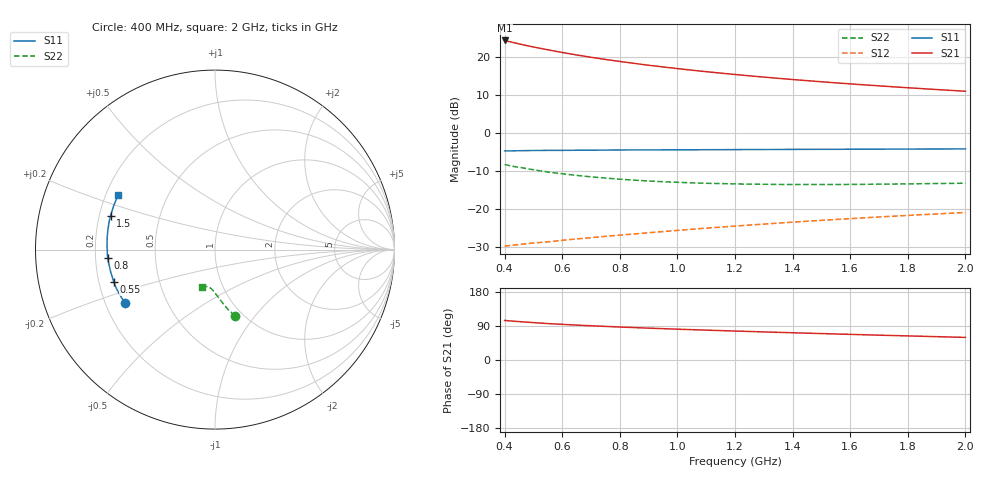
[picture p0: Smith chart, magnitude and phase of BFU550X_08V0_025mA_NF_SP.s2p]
! Filename:  P:\Prog\Test\Noise\ATS_data\Testdata_Net\BFU550X attenuator noise\BFU550X_APG2013_44_C05_08p0V_025mA_NF_CM01_D.sf
! Date/Time: Fri 26/Jul/2013 14:34:24
! BFU550X_APG2013_44_C05_08p0V_1to35mA_NF_CM01_Bias7_R.sf
! Noise Parameter Data File
! BFU550X_APG2013_44_C05_08p0V_1to35mA_NF_CM01
! Date/time: Mon Jul 22 10:19:05 2013
! VAR V_out= 8.001000
! VAR I_out= 24.995000
! VAR V_in= 0.796900
! VAR I_in= 0.264750
! Device data file deembeded for feedlines and parallel
! Original file: \BFU550X attenuator noise\BFU550X_APG2013_44_C05_08p0V_025mA_NF_CM01_R.sf
! Feed-files: PR005V01_100713_Feed1.s2p, PR005V01_100713_Feed2.s2p
! Parallel-file: PR005V01_100713_Par.s2p
# MHz S MA R 50
!  Freq-MHz  S11-mag  S11-arg  S21-mag  S21-arg  S12-mag  S12-arg  S22-mag  S22-arg
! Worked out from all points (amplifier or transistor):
!   37 points, 400 MHz to 2 GHz, reference 50 ohm
!   highest |S21| = 24.3 dB at 400 MHz (marker M1)
!   |S21| within 3 dB of that: start of sweep to 588.9 MHz
!   unconditionally stable (mu >= 1): 1.44 GHz to end of sweep
!   at 500 MHz: K = 0.66, MSG = 25.8 dB, |S12| = -28.9 dB
!   at 1.1 GHz: K = 0.95, MSG = 20.6 dB, |S12| = -25.0 dB
!   at 2 GHz: K = 1.04, MAG = 14.7 dB, |S12| = -20.9 dB
!   lowest NFmin = 1.10 dB at 480 MHz
!   S11 on the Smith chart (normalised r, x): 400 MHz: 0.28, -0.26; 550 MHz: 0.26, -0.15; 800 MHz: 0.25, -0.04; 1.5 GHz: 0.25, +0.15; 2 GHz: 0.25, +0.25
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400  0.5833 -149.1  16.48 104.3  0.03264 47.8  0.3859 -73.5
420  0.5829 -151.1  15.78 103.1  0.03332 48.1  0.3719 -74.8
440  0.5857 -153.0  15.16 101.9  0.03398 48.2  0.3593 -75.7
460  0.5869 -154.8  14.57 100.8  0.03465 48.3  0.3505 -76.9
500  0.5901 -158.1  13.53 98.7  0.03588 48.6  0.3301 -78.8
550  0.5922 -162.1  12.42 96.2  0.0372 49.4  0.3075 -81.0
600  0.5922 -165.1  11.46 94.1  0.03898 50.1  0.292 -82.8
650  0.5946 -168.1  10.62 92.1  0.04061 50.7  0.2777 -84.5
700  0.5953 -170.7  9.908 90.3  0.04222 51.5  0.2662 -86.0
750  0.5976 -173.1  9.278 88.7  0.04394 52.0  0.2563 -87.5
800  0.5995 -175.3  8.728 87.0  0.04559 52.6  0.2478 -88.9
850  0.6005 -177.5  8.235 85.5  0.0472 53.3  0.2405 -90.2
900  0.6004 -179.5  7.789 84.1  0.04899 53.9  0.2345 -91.4
950  0.6018 178.7  7.395 82.7  0.05075 54.4  0.2293 -92.5
1050  0.6031 175.2  6.706 80.1  0.05441 55.3  0.2217 -94.6
1100  0.6042 173.5  6.408 78.8  0.05628 55.6  0.2188 -95.5
1200  0.6062 170.4  5.885 76.4  0.05992 56.2  0.2148 -97.4
1350  0.6091 166.1  5.239 73.0  0.06557 56.9  0.2112 -100.0
1500  0.6113 162.1  4.722 69.7  0.0713 57.2  0.211 -102.4
1600  0.613 159.6  4.428 67.6  0.07504 57.3  0.2113 -103.8
1750  0.6151 155.9  4.052 64.6  0.08085 57.4  0.2139 -106.1
2000  0.6195 150.4  3.544 59.6  0.09038 57.1  0.2195 -109.5
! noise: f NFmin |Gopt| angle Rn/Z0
400  1.211  0.2937  -175.5  0.08
460  1.155  0.3332  -173.7  0.0681
600  1.169  0.3283  -172.3  0.0715
800  1.185  0.3507  -169.2  0.0676
1000  1.214  0.371  -166.3  0.0647
1200  1.239  0.3929  -163.8  0.0634
1400  1.252  0.3914  -160.1  0.072
1600  1.302  0.4157  -154.9  0.0739
1800  1.297  0.4165  -155.1  0.0742
2000  1.339  0.4335  -151.2  0.0828
